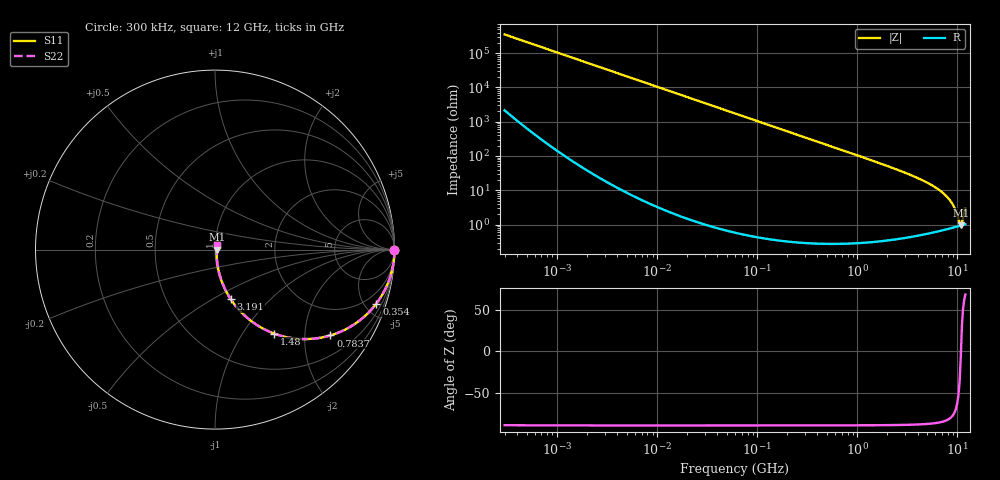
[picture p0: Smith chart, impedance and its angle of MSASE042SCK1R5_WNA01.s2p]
! MSASE042SCK1R5_WNA01  S-PARAMETER MODEL  ( General Type )
! Model Generated by TAIYO YUDEN Corporation (http://www.ty-top.com)
! Version 2.0
! TAIYO YUDEN Control No. 120810
! Copyright(c) 2011 TAIYO YUDEN CO.,LTD. All Rights Reserved.
! Product Description (link to TY-COMPAS)
! https://ds.yuden.co.jp/TYCOMPAS/or/detail?pn=MSASE042SCK1R5AWNA01&u=M
! Products Name : Multilayer Ceramic Capacitors
! Characteristics :
!  Capacitance : 1.5 pF , Rated Voltage : 16V , TCC : CK / C0K
!  Case Size : 0.4 x 0.2 / 0.016 x 0.008 [mm/inch] , Thickness : 0.2 / 0.008 [mm/inch]
!  (Conditions: Temperature = 25 degC , DC Bias Current/Voltage = 0A / 0V)
! External Node Assignments :
!  1  o---| |---o  2
! GND o---------o GND
! Frequency Range : 0.3MHz  -  12000MHz  [ 401 STEP ]
# MHz S RI R 50
! Freq[MHz].  S11 Real  S11 Imag  S21 Real  S21 Imag  S12 Real  S12 Imag  S22 Real  S22 Imag
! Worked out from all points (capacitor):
!   401 points, 300 kHz to 12 GHz, reference 50 ohm
!   read as one part in series: C = 1.51 pF near 316.3 kHz
!   lowest |Z| = 944 mohm at 10.79 GHz (marker M1)
!   series resonance near 10.83 GHz, so ESL is about 140 pH
!   S11 on the Smith chart (normalised r, x): 300 kHz: open; 354 MHz: 1.01, -5.97; 783.7 MHz: 1.01, -2.68; 1.48 GHz: 1.01, -1.40; 3.191 GHz: 1.01, -0.61; 12 GHz: 1.02, +0.05
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0.3  1 -0.000284  1.81e-06 0.000284  1.81e-06 0.000284  1 -0.000284
1.769972  1 -0.00167  4.13e-06 0.00167  4.13e-06 0.00167  1 -0.00167
10.44266  0.9999 -0.00988  0.000101 0.00988  0.000101 0.00988  0.9999 -0.00988
60  0.9968 -0.0566  0.00323 0.0566  0.00323 0.0566  0.9968 -0.0566
155.7172  0.9787 -0.1441  0.0213 0.1441  0.0213 0.1441  0.9787 -0.1441
353.9943  0.8988 -0.3011  0.1012 0.3011  0.1012 0.3011  0.8988 -0.3011
526.7124  0.8001 -0.3992  0.1999 0.3992  0.1999 0.3992  0.8001 -0.3992
783.7017  0.6428 -0.4782  0.3572 0.4782  0.3572 0.4782  0.6428 -0.4782
1076.992  0.4859 -0.4983  0.5141 0.4983  0.5141 0.4983  0.4859 -0.4983
1480.043  0.3303 -0.4681  0.6697 0.4681  0.6697 0.4681  0.3303 -0.4681
2088.533  0.1938 -0.3917  0.8062 0.3917  0.8062 0.3917  0.1938 -0.3917
3190.978  0.0872 -0.2753  0.9128 0.2753  0.9128 0.2753  0.0872 -0.2753
5140.631  0.03 -0.1542  0.97 0.1542  0.97 0.1542  0.03 -0.1542
7254.098  0.0132 -0.0794  0.9868 0.0794  0.9868 0.0794  0.0132 -0.0794
8064.993  0.0108 -0.058  0.9892 0.058  0.9892 0.058  0.0108 -0.058
8732.115  0.00968 -0.0424  0.9903 0.0424  0.9903 0.0424  0.00968 -0.0424
9454.42  0.0091 -0.0269  0.9909 0.0269  0.9909 0.0269  0.0091 -0.0269
10236.47  0.00905 -0.0117  0.991 0.0117  0.991 0.0117  0.00905 -0.0117
10511.28  0.00915 -0.00659  0.9909 0.00659  0.9909 0.00659  0.00915 -0.00659
10793.46  0.00931 -0.00097  0.9907 0.00097  0.9907 0.00097  0.00931 -0.00097
11083.22  0.00954 0.00581  0.9905 -0.00581  0.9905 -0.00581  0.00954 0.00581
12000  0.0109 0.0264  0.9891 -0.0264  0.9891 -0.0264  0.0109 0.0264
